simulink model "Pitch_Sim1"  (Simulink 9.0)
settings: Solver=ode45  StartTime=0.0  StopTime=120  RelTol=1e-3  EnableMultiTasking=on
InitFcn:
  | init_pitch;
StopFcn:
  | pl
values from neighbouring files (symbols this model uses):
  d2r = pi/180    (= 0.0174532925199)    [frequ.m]    (also in init_pitch.m; pl.m; init.m; freq.m)
undefined symbols (not defined in the file or in its folder): Ap, Bp, Cp, Dp, Kc

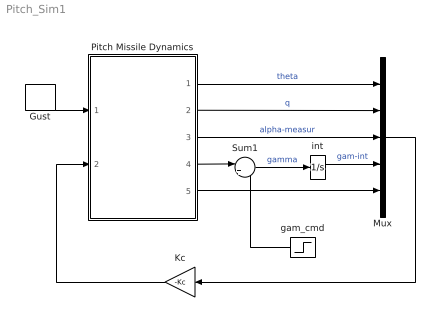
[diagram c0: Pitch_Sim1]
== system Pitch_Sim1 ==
  Gust : DiscretePulseGenerator  PulseType=Time based  Amplitude=30  Period=200  PulseWidth=2  PhaseDelay=20
  Kc : Gain  Gain=-Kc  Multiplication=Matrix(K*u)
  Mux : Mux  Inputs=5
  Pitch Missile Dynamics : Subsystem
  Sum1 : Sum  Inputs=|+-
  gam_cmd : Step  Time=0  After=1*d2r  SampleTime=0
  int : Integrator
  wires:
  Mux/1 -> Kc/1
  Pitch Missile Dynamics/1(theta) -> Mux/1  "theta"
  Pitch Missile Dynamics/2(q) -> Mux/2  "q"
  Pitch Missile Dynamics/4(gama) -> Sum1/1
  int/1 -> Mux/4  "gam-int"
  Sum1/1 -> int/1  "gamma"
  Kc/1 -> Pitch Missile Dynamics/2(Elevon)
  Pitch Missile Dynamics/5(delevn) -> Mux/5
  Pitch Missile Dynamics/3(alfav) -> Mux/3  "alpha-measur"
  Gust/1 -> Pitch Missile Dynamics/1(WGust)
  gam_cmd/1 -> Sum1/2

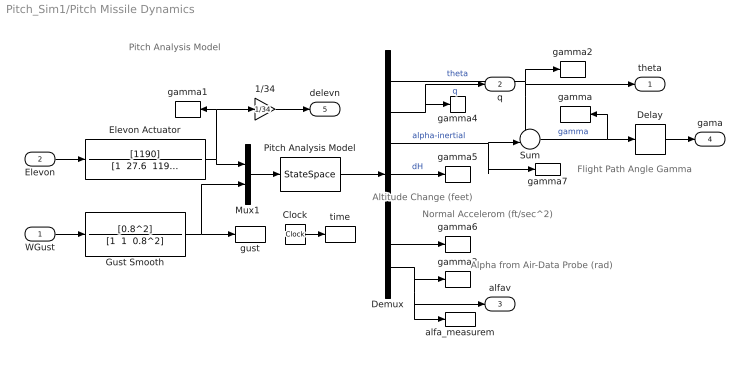
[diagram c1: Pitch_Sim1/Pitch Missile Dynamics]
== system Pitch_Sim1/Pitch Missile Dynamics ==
  note: Pitch Analysis Model
  note: Flight Path Angle Gamma
  note: Normal Accelerom (ft/sec^2)
  note: Alpha from Air-Data Probe (rad)
  note: Altitude Change (feet)
  WGust : Inport
  Elevon : Inport  Port=2
  1/34 : Gain  Gain=1/34
  Clock : Clock
  Delay : TransportDelay  DelayTime=0.7  PadeOrder=2
  Demux : Demux  Outputs=7
  Elevon Actuator : TransferFcn  Numerator=[1190]  Denominator="[1  27.6  1190]"
  Gust Smooth : TransferFcn  Numerator=[0.8^2]  Denominator="[1  1  0.8^2]"
  Mux1 : Mux  Inputs=2
  Pitch Analysis Model : StateSpace  A=Ap  B=Bp  C=Cp  D=Dp  InitialCondition=0
  Sum : Sum  Inputs=+-|
  alfa_measurem : ToWorkspace  VariableName=alfest  SampleTime=-1
  gamma : ToWorkspace  VariableName=Gam  SampleTime=-1
  gamma1 : ToWorkspace  VariableName=Elev  SampleTime=-1
  gamma2 : ToWorkspace  VariableName=Thet  SampleTime=-1
  gamma3 : ToWorkspace  VariableName=alfav  SampleTime=-1
  gamma4 : ToWorkspace  VariableName=q  SampleTime=-1
  gamma5 : ToWorkspace  VariableName=altit  SampleTime=-1
  gamma6 : ToWorkspace  VariableName=Az  SampleTime=-1
  gamma7 : ToWorkspace  VariableName=alfin  SampleTime=-1
  gust : ToWorkspace  VariableName=gust  SampleTime=-1
  time : ToWorkspace  VariableName=time  SampleTime=-1
  theta : Outport
  q : Outport  Port=2
  alfav : Outport  Port=3
  gama : Outport  Port=4
  delevn : Outport  Port=5
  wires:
  Demux/1 -> theta/1, Sum/1, gamma2/1  "theta"
  Delay/1 -> gama/1
  Pitch Analysis Model/1 -> Demux/1
  Demux/3 -> gamma7/1, Sum/2  "alpha-inertial"
  Demux/2 -> q/1, gamma4/1  "q"
  Clock/1 -> time/1
  Demux/4 -> gamma5/1  "dH"
  Demux/6 -> gamma6/1
  Sum/1 -> gamma/1, Delay/1  "gamma"
  Gust Smooth/1 -> gust/1, Mux1/2
  WGust/1 -> Gust Smooth/1
  Mux1/1 -> Pitch Analysis Model/1
  Elevon/1 -> Elevon Actuator/1
  Elevon Actuator/1 -> 1/34/1, gamma1/1, Mux1/1
  1/34/1 -> delevn/1
  Demux/7 -> alfa_measurem/1, alfav/1, gamma3/1
